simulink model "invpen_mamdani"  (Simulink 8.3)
settings: Solver=ode5  SolverMode=SingleTasking  StartTime=0.0  StopTime=20  FixedStep=.01  MaxStep=0.1  RelTol=1e-3  AbsTol=1e-6
PreLoadFcn:
  | init_m;
undefined symbols (not defined in the file or in its folder): g, init_cond, l, m, mc
libraries: fuzblock x1

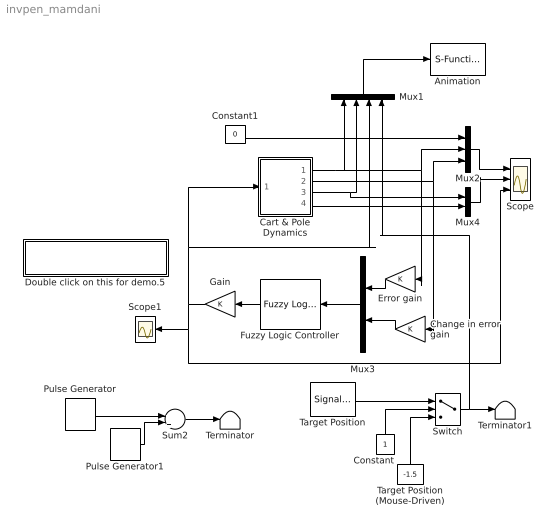
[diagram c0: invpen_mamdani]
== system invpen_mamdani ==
  Animation : S-Function  FunctionName=animcp  EnableBusSupport=off
  Cart & Pole Dynamics : Subsystem
  Change in error gain : Gain
  Constant : Constant
  Constant1 : Constant  Value=0
  Double click on this for demo.5 : Subsystem
  Error gain : Gain
  Fuzzy Logic Controller : fuzblock/Fuzzy Logic  Controller  fis=fismatrix
  Gain : Gain
  Mux1 : Mux
  Mux2 : Mux  Inputs=3
  Mux3 : Mux  Inputs=2
  Mux4 : Mux  Inputs=2
  Pulse Generator : DiscretePulseGenerator  PulseType=Time based  Amplitude=10  Period=10  PulseWidth=0.2  PhaseDelay=1
  Pulse Generator1 : DiscretePulseGenerator  PulseType=Time based  Amplitude=-10  Period=10  PulseWidth=0.2  PhaseDelay=6
  Scope : Scope  NumInputPorts=3
  Scope1 : Scope
  Sum2 : Sum  Inputs=+|+
  Switch : Switch
  Target Position : SignalGenerator  WaveForm=sawtooth  Amplitude=0.05  Frequency=3*0.628320  Units=rad/sec
  Target Position (Mouse-Driven) : Constant  Value=-1.5
  Terminator : Terminator
  Terminator1 : Terminator
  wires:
  Cart & Pole Dynamics/4(out_4) -> Mux4/2
  Mux3/1 -> Fuzzy Logic Controller/1
  Mux2/1 -> Scope/1
  Mux4/1 -> Scope/2
  Cart & Pole Dynamics/3(out_3) -> Mux4/1, Mux1/2
  Cart & Pole Dynamics/2(out_2) -> Mux2/3, Change in error gain/1
  Fuzzy Logic Controller/1 -> Gain/1
  Pulse Generator/1 -> Sum2/1
  Pulse Generator1/1 -> Sum2/2
  Target Position/1 -> Switch/1
  Constant/1 -> Switch/2
  Target Position (Mouse-Driven)/1 -> Switch/3
  Gain/1 -> Scope/3, Scope1/1, Mux1/3, Cart & Pole Dynamics/1(in_1)
  Constant1/1 -> Mux2/1
  Error gain/1 -> Mux3/1
  Change in error gain/1 -> Mux3/2
  Sum2/1 -> Terminator/1
  Switch/1 -> Terminator1/1, Mux1/4
  Cart & Pole Dynamics/1(out_1) -> Error gain/1, Mux2/2, Mux1/1
  Mux1/1 -> Animation/1

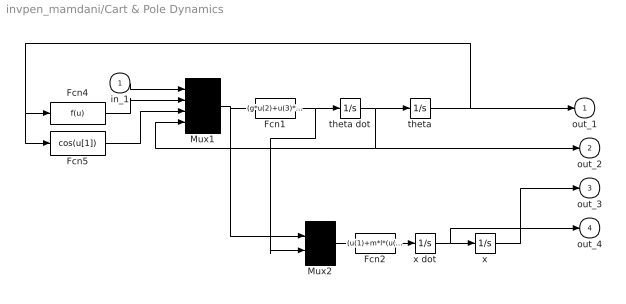
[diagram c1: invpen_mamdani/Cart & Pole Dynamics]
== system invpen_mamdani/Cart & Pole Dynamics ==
  in_1 : Inport
  Fcn1 : Fcn  Expr=(g*u(2)+u(3)*((-u(1)-m*l*u(4)*u(4)*u(2))/(mc+m)))/(l*(4/3-(m*u(3)*u(3))/(mc+m)))
  Fcn2 : Fcn  Expr=(u(1)+m*l*(u(4)*u(4)*u(2)-u(5)*u(3)))/(mc+m)
  Fcn4 : Fcn
  Fcn5 : Fcn  Expr=cos(u[1])
  Mux1 : Mux
  Mux2 : Mux  Inputs=[4,1]
  theta : Integrator  InitialCondition=init_cond(1)
  theta dot : Integrator  InitialCondition=init_cond(2)
  x : Integrator  InitialCondition=init_cond(3)
  x dot : Integrator  InitialCondition=init_cond(4)
  out_1 : Outport  InitialOutput=0
  out_2 : Outport  Port=2  InitialOutput=0
  out_3 : Outport  Port=3  InitialOutput=0
  out_4 : Outport  Port=4  InitialOutput=0
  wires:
  in_1/1 -> Mux1/1
  x/1 -> out_3/1
  x dot/1 -> out_4/1, x/1
  Mux1/1 -> Fcn1/1, Mux2/1
  Mux2/1 -> Fcn2/1
  Fcn2/1 -> x dot/1
  Fcn1/1 -> Mux2/2, theta dot/1
  theta dot/1 -> Mux1/4, out_2/1, theta/1
  Fcn4/1 -> Mux1/2
  Fcn5/1 -> Mux1/3
  theta/1 -> Fcn4/1, Fcn5/1, out_1/1

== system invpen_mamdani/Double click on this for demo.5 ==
